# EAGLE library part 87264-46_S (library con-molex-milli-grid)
RECEPTACAL
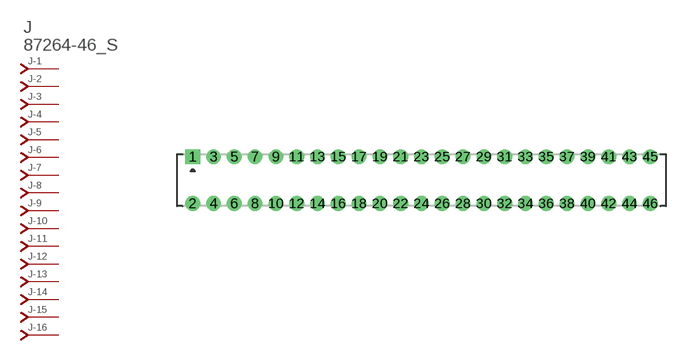
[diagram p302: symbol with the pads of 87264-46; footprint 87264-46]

Designator prefix J; gates -1=J-NV -2=J-N -3=J-N -4=J-N -5=J-N -6=J-N -7=J-N -8=J-N -9=J-N -10=J-N -11=J-N -12=J-N -13=J-N -14=J-N -15=J-N -16=J-N -17=J-N -18=J-N -19=J-N -20=J-N -21=J-N -22=J-N -23=J-N -24=J-N -25=J-N -26=J-N -27=J-N -28=J-N -29=J-N -30=J-N -31=J-N -32=J-N -33=J-N -34=J-N -35=J-N -36=J-N -37=J-N -38=J-N -39=J-N -40=J-N -41=J-N -42=J-N -43=J-N -44=J-N -45=J-N -46=J-N

## 87264-46_S  [87264-46]
1  -1:J  pas
2  -2:J  pas
3  -3:J  pas
4  -4:J  pas
5  -5:J  pas
6  -6:J  pas
7  -7:J  pas
8  -8:J  pas
9  -9:J  pas
10  -10:J  pas
11  -11:J  pas
12  -12:J  pas
13  -13:J  pas
14  -14:J  pas
15  -15:J  pas
16  -16:J  pas
17  -17:J  pas
18  -18:J  pas
19  -19:J  pas
20  -20:J  pas
21  -21:J  pas
22  -22:J  pas
23  -23:J  pas
24  -24:J  pas
25  -25:J  pas
26  -26:J  pas
27  -27:J  pas
28  -28:J  pas
29  -29:J  pas
30  -30:J  pas
31  -31:J  pas
32  -32:J  pas
33  -33:J  pas
34  -34:J  pas
35  -35:J  pas
36  -36:J  pas
37  -37:J  pas
38  -38:J  pas
39  -39:J  pas
40  -40:J  pas
41  -41:J  pas
42  -42:J  pas
43  -43:J  pas
44  -44:J  pas
45  -45:J  pas
46  -46:J  pas

## Footprint 87264-46 (pad centres in mm)
RECEPTACAL Dual Row, Side Entry
drill 0.914 square: 1 -22,2.25
drill 0.914: 2 -22,-2.25; 3 -20,2.25; 4 -20,-2.25; 5 -18,2.25; 6 -18,-2.25; 7 -16,2.25; 8 -16,-2.25; 9 -14,2.25; 10 -14,-2.25; 11 -12,2.25; 12 -12,-2.25; 13 -10,2.25; 14 -10,-2.25; 15 -8,2.25; 16 -8,-2.25; 17 -6,2.25; 18 -6,-2.25; 19 -4,2.25; 20 -4,-2.25; 21 -2,2.25; 22 -2,-2.25; 23 0,2.25; 24 0,-2.25; 25 2,2.25; 26 2,-2.25; 27 4,2.25; 28 4,-2.25; 29 6,2.25; 30 6,-2.25; 31 8,2.25; 32 8,-2.25; 33 10,2.25; 34 10,-2.25; 35 12,2.25; 36 12,-2.25; 37 14,2.25; 38 14,-2.25; 39 16,2.25; 40 16,-2.25; 41 18,2.25; 42 18,-2.25; 43 20,2.25; 44 20,-2.25; 45 22,2.25; 46 22,-2.25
